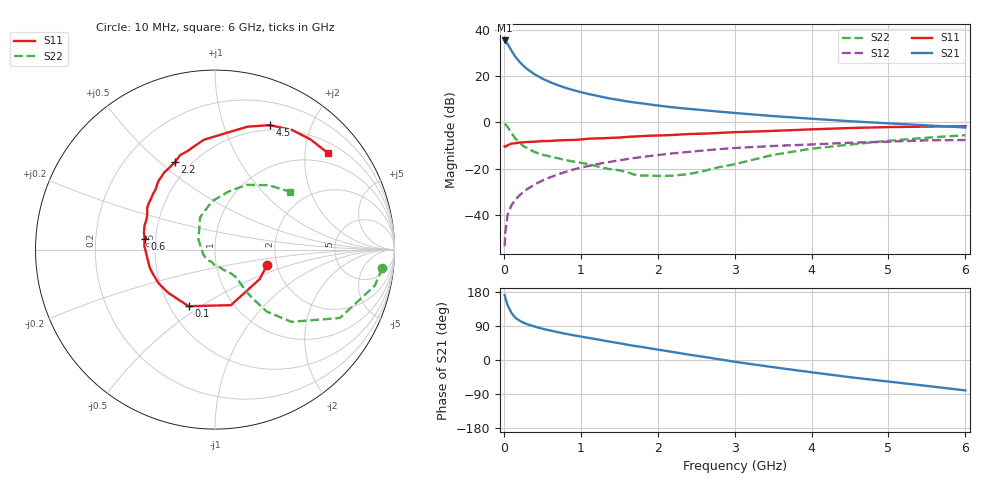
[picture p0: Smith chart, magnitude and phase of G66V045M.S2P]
! SIEMENS Small Signal Semiconductors
! BFG193
! Si NPN RF Bipolar Junction Transistor in SOT223
! VCE = 6 V  IC = 45 mA
! Common Emitter S-Parameters:  August  1996
# GHz  S  MA  R  50
!  f  S11  S21  S12  S22
! GHz  MAG  ANG  MAG  ANG  MAG  ANG  MAG  ANG
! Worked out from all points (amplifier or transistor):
!   36 points, 10 MHz to 6 GHz, reference 50 ohm
!   highest |S21| = 35.5 dB at 10 MHz (marker M1)
!   |S21| within 3 dB of that: start of sweep to 74.47 MHz
!   unconditionally stable (mu >= 1): 487.1 MHz to 2.377 GHz
!   at 250 MHz: K = 0.89, MSG = 27.4 dB, |S12| = -30.2 dB
!   at 1.4 GHz: K = 1.04, MAG = 12.4 dB, |S12| = -17.0 dB
!   at 6 GHz: K = 0.89, MSG = 2.7 dB, |S12| = -7.6 dB
!   S11 on the Smith chart (normalised r, x): 10 MHz: 1.77, -0.34; 100 MHz: 0.62, -0.45; 600 MHz: 0.43, +0.06; 2.2 GHz: 0.41, +0.56; 4.5 GHz: 0.44, +1.44; 6 GHz: 0.73, +2.51
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0.01  0.3021 -16.8  59.42 171.3  0.0021 88.8  0.9373 -6.3
0.02  0.2982 -33.6  57.74 164.0  0.0043 80.2  0.9127 -12.7
0.05  0.322 -74.0  49.33 143.9  0.0102 72.1  0.7935 -28.7
0.1  0.348 -115.0  35.63 124.0  0.0163 66.3  0.5857 -43.4
0.15  0.3547 -137.1  26.35 111.4  0.0212 65.4  0.4499 -50.1
0.2  0.3663 -149.1  20.88 104.4  0.0261 67.0  0.3708 -51.7
0.25  0.3712 -158.4  17.07 98.8  0.031 67.0  0.3122 -52.9
0.3  0.3775 -164.8  14.45 94.7  0.0357 68.1  0.2787 -53.2
0.4  0.3823 -175.3  11.03 88.4  0.0452 68.1  0.2294 -52.9
0.5  0.3944 177.1  8.88 82.6  0.055 67.7  0.2005 -52.5
0.6  0.397 171.3  7.464 77.9  0.0647 66.8  0.1834 -53.5
0.7  0.407 166.6  6.422 73.5  0.0751 65.8  0.1683 -55.3
0.8  0.4151 161.1  5.62 69.3  0.0847 64.0  0.1533 -57.1
1.1  0.4435 148.5  4.126 58.4  0.1141 58.9  0.1246 -66.7
1.4  0.4639 138.0  3.249 47.7  0.142 52.7  0.0965 -80.6
1.6  0.4855 131.6  2.856 40.6  0.161 48.2  0.0843 -93.7
2.2  0.5354 114.7  2.123 21.0  0.2143 34.8  0.0704 -155.4
2.8  0.5929 100.1  1.713 1.9  0.2645 20.9  0.1079 148.6
3.5  0.6555 83.9  1.373 -18.9  0.3093 3.8  0.1987 114.6
4.5  0.7573 66.3  1.063 -45.4  0.3639 -16.1  0.3322 76.9
5.5  0.8123 49.1  0.865 -68.4  0.4098 -39.3  0.4674 50.1
6  0.8273 40.7  0.776 -80.3  0.416 -52.7  0.5294 37.4
